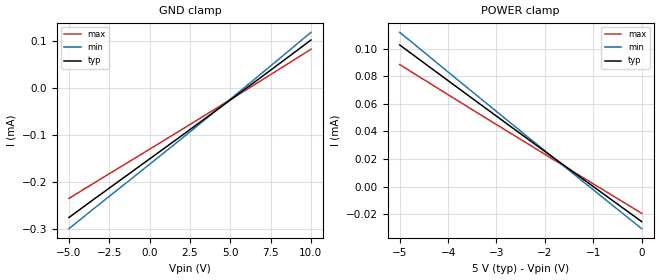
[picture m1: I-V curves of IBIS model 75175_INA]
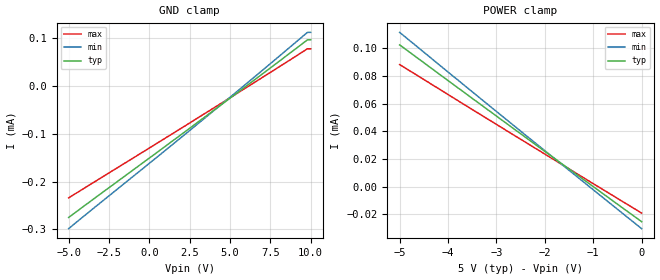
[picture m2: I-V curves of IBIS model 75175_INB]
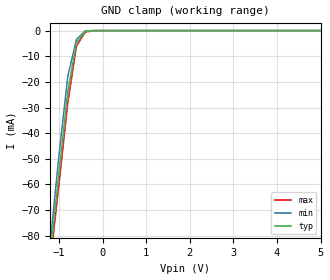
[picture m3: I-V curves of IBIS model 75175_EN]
|   TEXAS INSTRUMENTS INCORPORATED
|   Standard Linear and Logic Group
|   IBIS Model of SN75175
|   QUADRUPLE DIFFERENTIAL LINE RECEIVERS
|   SOIC 16-pin (D), PDIP 16-pin (N), SOP 16-pin (NS),
[IBIS Ver]   3.2
[Comment char] |_char
[File Name]   sn75175.ibs
[File Rev]   1.1 | c_die
[Date]   09/09/2005
[Source]   File originated at Texas Instruments, Inc
[Notes]   The following is a sample IBIS file for the SN75175.
   - FILE REV HISTORY
   - 1.1 Release IBIS file on 09/23/05
   - All test data contained in this file are derived from
   actual measurement.
   - The measurement used NS package.
   - We have data across voltage and temperature, but not across
   process.
   - Due to series resistor at the inputs, Pwr_clamp
   and Gnd_Clamp has non-zero current at the zero voltage levels
   - We removed the Pwr_Clamp data from the EN model since the
   current was insignificant
   - File created by TIJ SLL Product Engineering.
[Disclaimer] Property of Texas Instruments Incorporated.  Unauthorized
   reproduction and/or distribution is strictly prohibited.
   This product is protected under copyright law.
   Created 2000, (C) Copyright 2000, Texas Instruments Inc.,
   All Rights Reserved.
   UNLESS THERE IS A SIGNED, WRITTEN AGREEMENT TO THE
   CONTRARY, TEXAS INSTRUMENTS () IS PROVIDING THE IBIS
   MODELS  AND WITHOUT ANY WARRANTY, EXPRESSED OR
   IMPLIED.  TI assumes no liability for:
   1) the accuracy of the IBIS models provided to your
   company;
   2) the proper functioning of these IBIS Models in your
   design or for any resulting applications; or
   3) infringement of patents, copyrights or intellectual
   property rights resulting from your use of these IBIS
   models.
   TI provides IBIS Models as a service to our customers.
   You and your company shall not distribute, sell or give
   these models to anyone else without prior written
   permission from TI.
   TI reserves the right to make changes to our products or
   to discontinue any semiconductor product or service
   without notice, and advises our customers to obtain the
   latest version of relevant information to verify, before
   placing orders, that the information being relied on is
   current.
   Please be aware that your receipt and use of the IBIS
   information provided shall serve as acceptance of these
   terms and conditions.  If you do not accept these terms,
   you should return or destroy the IBIS models and any
   other accompanying information immediately.
|   Component 75175_D
[Component]   75175_D
[Manufacturer]  Texas Instruments, Inc.
[Package]
|   typ   min   max
R_pkg   0.039   0.028   0.049
L_pkg   3.453nH   2.350nH   4.375nH
C_pkg   0.521pF   0.254pF   0.708pF
[Pin]   signal_name   model_name   R_pin   L_pin   C_pin
1   1B   75175_INB   0.042   4.336nH   0.703pF
2   1A   75175_INA   0.049   3.778nH   0.634pF
3   1Y   75175_OUT   0.028   3.449nH   0.518pF
4   1,2EN   75175_EN   0.029   2.393nH   0.254pF
5   2Y   75175_OUT   0.028   2.350nH   0.264pF
6   2A   75175_INA   0.048   3.312nH   0.483pF
7   2B   75175_INB   0.043   3.629nH   0.604pF
8   GND   GND   0.044   4.375nH   0.708pF
9   3B   75175_INB   0.042   4.336nH   0.703pF
10   3A   75175_INA   0.049   3.778nH   0.634pF
11   3Y   75175_OUT   0.028   3.449nH   0.518pF
12   3,4EN   75175_EN   0.029   2.393nH   0.255pF
13   4Y   75175_OUT   0.028   2.350nH   0.264pF
14   4A   75175_INA   0.048   3.312nH   0.483pF
15   4B   75175_INB   0.043   3.629nH   0.604pF
16   VCC   POWER   0.044   4.375nH   0.708pF
| Component 75175_N
[Component]   75175_N
[Manufacturer]  Texas Instruments, Inc.
[Package]
|   typ   min   max
R_pkg   5.600e-02   5.200e-02   6.300e-02
L_pkg   7.637e-09   5.451e-09   1.053e-08
C_pkg   5.280e-13   3.350e-13   8.930e-13
[Pin]   signal_name   model_name   R_pin   L_pin   C_pin
1   1B   75175_INB   5.800e-02   1.053e-08   8.920e-13
2   1A   75175_INA   6.200e-02   8.759e-09   5.350e-13
3   1Y   75175_OUT   5.200e-02   7.146e-09   3.870e-13
4   1,2EN   75175_EN   5.300e-02   5.451e-09   4.080e-13
5   2Y   75175_OUT   5.300e-02   5.513e-09   3.700e-13
6   2A   75175_INA   5.300e-02   6.304e-09   3.360e-13
7   2B   75175_INB   5.700e-02   7.830e-09   5.030e-13
8   GND   GND   5.600e-02   9.581e-09   8.050e-13
9   3B   75175_INB   5.800e-02   9.603e-09   8.070e-13
10   3A   75175_INA   6.200e-02   7.864e-09   5.030e-13
11   3Y   75175_OUT   5.200e-02   6.295e-09   3.350e-13
12   3,4EN   75175_EN   5.300e-02   5.499e-09   3.560e-13
13   4Y   75175_OUT   5.300e-02   5.452e-09   4.040e-13
14   4A   75175_INA   5.300e-02   7.156e-09   3.870e-13
15   4B   75175_INB   6.300e-02   8.740e-09   5.340e-13
16   VCC   POWER   5.600e-02   1.048e-08   8.930e-13
|   Component 75A175_NS
[Component]   75175_NS
[Manufacturer]  Texas Instruments, Inc.
[Package]
|   typ   min   max
R_pkg   0.042   0.035   0.049
L_pkg   3.147nH   2.164nH   4.219nH
C_pkg   0.404pF   0.241pF   0.562pF
[Pin]   signal_name   model_name   R_pin   L_pin   C_pin
1   1B   75175_INB   0.049   4.215nH   0.562pF
2   1A   75175_INA   0.046   3.675nH   0.480pF
3   1Y   75175_OUT   0.037   2.527nH   0.332pF
4   1,2EN   75175_EN   0.035   2.164nH   0.241pF
5   2Y   75175_OUT   0.035   2.164nH   0.241pF
6   2A   75175_INA   0.037   2.527nH   0.332pF
7   2B   75175_INB   0.046   3.675nH   0.480pF
8   GND   GND   0.049   4.215nH   0.562pF
9   3B   75175_INB   0.049   4.219nH   0.562pF
10   3A   75175_INA   0.046   3.679nH   0.480pF
11   3Y   75175_OUT   0.037   2.531nH   0.333pF
12   3,4EN   75175_EN   0.035   2.168nH   0.241pF
13   4Y   75175_OUT   0.035   2.168nH   0.241pF
14   4A   75175_INA   0.037   2.531nH   0.333pF
15   4B   75175_INB   0.046   3.679nH   0.480pF
16   VCC   POWER   0.049   4.219nH   0.562pF
[Diff_pin]   inv_pin   vdiff   tdelay_typ   tdelay_min   tdelay_max
| The 'xA' pin is Diff_pin and the 'xB' pin is the inv_pin
2   1   200mV   0 0 0   | Vth  +/-200mV
6   7   200mV   0 0 0
10   9   200mV   0 0 0
14   15   200mV   0 0 0
| Models and submodels in the file (4): 75175_INA (Input), 75175_INB (Input), 75175_EN (Input), 75175_OUT (3-state)
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|   Model 75175_INA
[Model]   75175_INA
Model_type  Input
Polarity   Non-Inverting
Vinl = 0.8
Vinh = 2.0
| variable   typ   min   max
C_comp   2.625pf   2.505pf   2.863pf
[Temperature Range]   25   0   70
[Voltage Range]   5.0   4.75   5.25
[GND Clamp]
|   Voltage   I(typ)   I(min)   I(max)
-5V       -275.8uA   -299.7uA   -235.2uA
3.4V      -65.73uA   -68.22uA   -58.53uA
6.4V      10.2uA     16.04uA    5.221uA
10V       102.6uA    118.8uA    82.93uA
[POWER Clamp]
|   Voltage   I(typ)   I(min)   I(max)
-5V       102.6uA    111.7uA    88.39uA
-2.7V     43.36uA    45.84uA    38.5uA
-1.5V     12.78uA    11.78uA    12.73uA
0V        -25.3uA    -30.42uA   -19.27uA
|   Model 75175_INB
[Model]   75175_INB
Model_type  Input
Polarity   Inverting
Vinl = 0.8
Vinh = 2.0
| variable   typ   min   max
C_comp   2.947pf   2.780pf   3.188pf
[Temperature Range]   25   0   70
[Voltage Range]   5.0   4.75   5.25
[GND Clamp]
|   Voltage   I(typ)   I(min)   I(max)
-5V       -275.5uA   -298.9uA   -234.4uA
2.8V      -80.82uA   -84.72uA   -70.93uA
9.8V      97.27uA    112.8uA    78.47uA
10V       97.27uA    112.8uA    78.47uA
[POWER Clamp]
|   Voltage   I(typ)   I(min)   I(max)
-5V       102.4uA    111.4uA    88.16uA
-3.5V     63.77uA    68.53uA    55.73uA
-2.4V     35.67uA    37.25uA    32.11uA
0V        -25.3uA    -30.33uA   -19.1uA
|   Model 75A175_EN
[Model]   75175_EN
Model_type  Input
Polarity   Non-Inverting
Vinl = 0.8
Vinh = 2.0
| variable   typ   min   max
C_comp   2.630pf   2.491pf   3.002pf
[Temperature Range]   25   0   70
[Voltage Range]   5.0   4.75   5.25
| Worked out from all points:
|   GND clamp passes 1 mA (typ) near -0.43 V on its own axis
[GND Clamp]
|   Voltage   I(typ)   I(min)   I(max)
-5V       -673.5mA   -715.4mA   -647.1mA
-1.2V     -87.16mA   -82.51mA   -90.12mA
-1V       -55.43mA   -48.52mA   -59.96mA
-800mV    -23.96mA   -17.97mA   -28.42mA
-600mV    -4.767mA   -3.425mA   -6.091mA
-400mV    -315.1uA   -73.77uA   -589uA
-200mV    -12.43uA   -11.84uA   -14.96uA
5V        456.5nA    393.5nA    516.5nA
